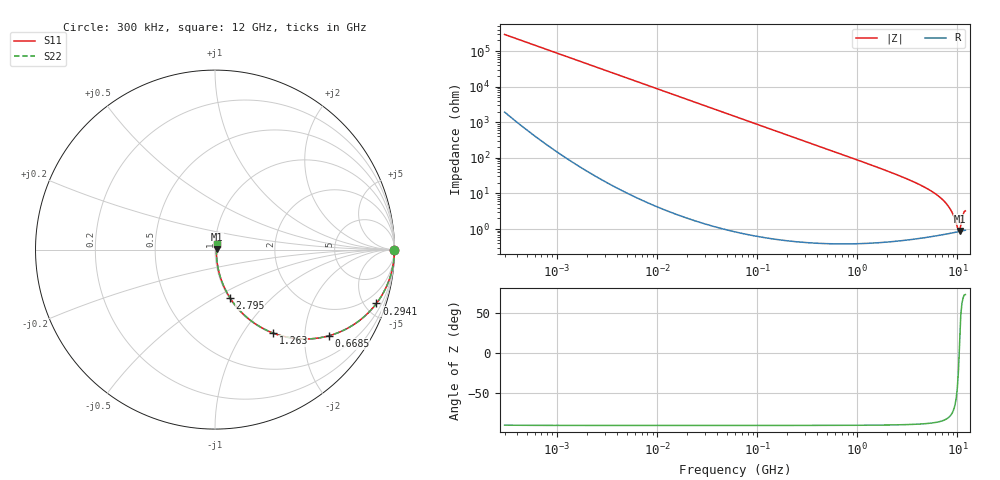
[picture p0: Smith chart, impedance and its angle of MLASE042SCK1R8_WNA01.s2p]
! MLASE042SCK1R8_WNA01  S-PARAMETER MODEL  ( General Type )
! Model Generated by TAIYO YUDEN Corporation (http://www.ty-top.com)
! Version 1.0
! TAIYO YUDEN Control No. 120810
! Copyright(c) 2012 TAIYO YUDEN CO.,LTD. All Rights Reserved.
! Product Description (link to TY-COMPAS)
! https://ds.yuden.co.jp/TYCOMPAS/or/detail?pn=MLASE042SCK1R8AWNA01&u=M
! Products Name : Multilayer Ceramic Capacitors
! Characteristics :
!  Capacitance : 1.8 pF , Rated Voltage : 16V , TCC : CK / C0K
!  Case Size : 0.4 x 0.2 / 0.016 x 0.008 [mm/inch] , Thickness : 0.2 / 0.008 [mm/inch]
!  (Conditions: Temperature = 25 degC , DC Bias Current/Voltage = 0A / 0V)
! External Node Assignments :
!  1  o---| |---o  2
! GND o---------o GND
! Frequency Range : 0.3MHz  -  12000MHz  [ 401 STEP ]
# MHz S RI R 50
! Freq[MHz].  S11 Real  S11 Imag  S21 Real  S21 Imag  S12 Real  S12 Imag  S22 Real  S22 Imag
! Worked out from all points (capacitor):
!   401 points, 300 kHz to 12 GHz, reference 50 ohm
!   read as one part in series: C = 1.8 pF near 316.3 kHz
!   lowest |Z| = 881 mohm at 10.51 GHz (marker M1)
!   series resonance near 10.4 GHz, so ESL is about 130 pH
!   S11 on the Smith chart (normalised r, x): 300 kHz: open; 294.1 MHz: 1.01, -5.99; 668.5 MHz: 1.01, -2.63; 1.263 GHz: 1.01, -1.38; 2.795 GHz: 1.01, -0.59; 12 GHz: 1.02, +0.06
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0.3  1 -0.00034  2.35e-06 0.00034  2.35e-06 0.00034  1 -0.00034
1.769972  1 -0.00201  6.11e-06 0.00201  6.11e-06 0.00201  1 -0.00201
10.44266  0.9999 -0.0118  0.000146 0.0118  0.000146 0.0118  0.9999 -0.0118
60  0.9954 -0.0677  0.00465 0.0677  0.00465 0.0677  0.9954 -0.0677
140.0606  0.9753 -0.1549  0.0247 0.1549  0.0247 0.1549  0.9753 -0.1549
294.0765  0.8994 -0.3  0.1006 0.3  0.1006 0.3  0.8994 -0.3
353.9943  0.8605 -0.3456  0.1395 0.3456  0.1395 0.3456  0.8605 -0.3456
668.5285  0.6328 -0.4806  0.3672 0.4806  0.3672 0.4806  0.6328 -0.4806
918.7169  0.4758 -0.4974  0.5242 0.4974  0.5242 0.4974  0.4758 -0.4974
1262.535  0.3224 -0.4645  0.6776 0.4645  0.6776 0.4645  0.3224 -0.4645
2088.533  0.1438 -0.3455  0.8562 0.3455  0.8562 0.3455  0.1438 -0.3455
2795.104  0.0826 -0.2674  0.9174 0.2674  0.9174 0.2674  0.0826 -0.2674
4747.894  0.0266 -0.1426  0.9734 0.1426  0.9734 0.1426  0.0266 -0.1426
6699.894  0.0125 -0.0759  0.9875 0.0759  0.9875 0.0759  0.0125 -0.0759
8281.503  0.00894 -0.0388  0.9911 0.0388  0.9911 0.0388  0.00894 -0.0388
8966.534  0.00839 -0.0253  0.9916 0.0253  0.9916 0.0253  0.00839 -0.0253
9968.853  0.00827 -0.00762  0.9917 0.00762  0.9917 0.00762  0.00827 -0.00762
10236.47  0.00835 -0.00323  0.9916 0.00323  0.9916 0.00323  0.00835 -0.00323
10511.28  0.00847 0.00211  0.9915 -0.00211  0.9915 -0.00211  0.00847 0.00211
10793.46  0.00869 0.0095  0.9913 -0.0095  0.9913 -0.0095  0.00869 0.0095
11380.75  0.00942 0.0232  0.9906 -0.0232  0.9906 -0.0232  0.00942 0.0232
12000  0.0101 0.0304  0.9899 -0.0304  0.9899 -0.0304  0.0101 0.0304
